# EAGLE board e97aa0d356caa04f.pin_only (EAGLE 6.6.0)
REV: D

Size 50.8 x 22.86 mm. Coordinates in mm from the lower left corner, seen from the top.
Outline: 0,20.95 0,1.91 arc90 1.91,0 48.9,0 arc90 50.8,1.91 50.8,20.95 arc90 48.9,22.86 1.91,22.86 arc90 0,20.95
Copper layers (1*16): Top 0.035mm / dielectric 1.5mm / Bottom 0.035mm
Design rules "adafruit *": minimum track width 10mil, minimum drill 15.5mil, track to track 8mil, track to pad 8mil, pad to pad 8mil, via to via 8mil, smd to smd 8mil, copper to edge 10mil, drill to drill 8mil, minimum pad ring 10mil, minimum via ring 8mil, stop-mask expansion 2mil, vias tented up to drill 20mil, thermal gap 10mil

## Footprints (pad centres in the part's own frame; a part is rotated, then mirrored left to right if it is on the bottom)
0805-NO = smd 1.3 x 1.5: 1 -0.95,0; 2 0.95,0
0805_10MGAP = smd 1.2 x 1.5: 1 -1.05,0; 2 1.05,0
1X14-CB = drill 1.016 pad 1.778: 1 -16.51,0; 2 -13.97,0; 3 -11.43,0; 4 -8.89,0; 5 -6.35,0; 6 -3.81,0; 7 -1.27,0; 8 1.27,0; 9 3.81,0; 10 6.35,0; 11 8.89,0; 12 11.43,0; 13 13.97,0; 14 16.51,0
SOD-323 = smd 1.35 x 0.8: A 1.27,0; C -1.27,0
SOD-123 = smd 1.4 x 1.4: A 1.85,0; C -1.85,0
_0805MP = smd 1.2 x 1.3: 1 -1.016,0; 2 1.016,0
FIDUCIAL_1MM = smd 1 x 1: 1 0,0
CHIPLED_0805_NOOUTLINE = smd 1.2 x 1.2: A 0,-1.05; C 0,1.05
TERMBLOCK_1X2-3.5MM = drill 1 pad 2.184: 1 1.8,0; 2 -1.7,0
RESPACK_4X0603 = smd 0.45 x 0.9: 1 -1.3,-0.85; 2 -0.4,-0.85; 3 0.4,-0.85; 4 1.3,-0.85; 5 1.3,0.85; 6 0.4,0.85; 7 -0.4,0.85; 8 -1.3,0.85
SOLDERJUMPER_ARROW_NOPASTE = smd 0.762 x 1.524: 1 -1.016,0; 2 1.016,0
SOLDERJUMPER_CLOSEDWIRE = smd 1.168 x 1.6: 1 -0.762,0; 2 0.762,0 | smd 0.635 x 0.203: WIRE 0,0
B1,27 = smd 1.27 x 1.27: TP 0,0
SOIC8_208MIL = smd 0.6 x 2.2: 1 -1.905,-3.315; 2 -0.635,-3.315; 3 0.635,-3.315; 4 1.905,-3.315; 5 1.905,3.315; 6 0.635,3.315; 7 -0.635,3.315; 8 -1.905,3.315
LQFP48 = smd 1.1 x 0.285: 1 -4.2,2.75; 2 -4.2,2.25; 3 -4.2,1.75; 4 -4.2,1.25; 5 -4.2,0.75; 6 -4.2,0.25; 7 -4.2,-0.25; 8 -4.2,-0.75; 9 -4.2,-1.25; 10 -4.2,-1.75; 11 -4.2,-2.25; 12 -4.2,-2.75; 25 4.2,-2.75; 26 4.2,-2.25; 27 4.2,-1.75; 28 4.2,-1.25; 29 4.2,-0.75; 30 4.2,-0.25; 31 4.2,0.25; 32 4.2,0.75; 33 4.2,1.25; 34 4.2,1.75; 35 4.2,2.25; 36 4.2,2.75 | smd 0.285 x 1.1: 13 -2.75,-4.2; 14 -2.25,-4.2; 15 -1.75,-4.2; 16 -1.25,-4.2; 17 -0.75,-4.2; 18 -0.25,-4.2; 19 0.25,-4.2; 20 0.75,-4.2; 21 1.25,-4.2; 22 1.75,-4.2; 23 2.25,-4.2; 24 2.75,-4.2; 37 2.75,4.2; 38 2.25,4.2; 39 1.75,4.2; 40 1.25,4.2; 41 0.75,4.2; 42 0.25,4.2; 43 -0.25,4.2; 44 -0.75,4.2; 45 -1.25,4.2; 46 -1.75,4.2; 47 -2.25,4.2 | smd 0.28 x 1.1: 48 -2.75,4.2
WQFN20 = smd 0.28 x 0.75: 1 -1,-1.975; 2 -0.5,-1.975; 3 0,-1.975; 4 0.5,-1.975; 5 1,-1.975; 11 1,1.975; 12 0.5,1.975; 13 0,1.975; 14 -0.5,1.975; 15 -1,1.975 | smd 0.75 x 0.28: 6 1.975,-1; 7 1.975,-0.5; 8 1.975,0; 9 1.975,0.5; 10 1.975,1; 16 -1.975,1; 17 -1.975,0.5; 18 -1.975,0; 19 -1.975,-0.5; 20 -1.975,-1 | smd 2.45 x 2.45: 21 0,0
MOUNTINGHOLE_2.5_PLATED = drill 2.5 pad 3.2: P$1 0,0
4UCONN_20329 = smd 1 x 2: BASE@1 -0.75,-2; BASE@2 0.75,-2 | smd 0.4 x 1.35: D+ 0,0.775; D- -0.65,0.775; GND 1.3,0.775; ID 0.65,0.775; VBUS -1.3,0.775 | drill 0.7 offset: SPRT@1 -3.3,0.9; SPRT@2 3.3,0.9 | drill 0.6 pad 2.5 square: SPRT@3 -3.6,-1.9; SPRT@4 3.6,-1.9 | hole 0.7: -1.95,0; 1.95,0
JSTPH2 = smd 1 x 4.6: 1 -1,-3.7; 2 1,-3.7 | smd 1.6 x 3.4: NC1 -3.4,1.5; NC2 3.4,1.5
RESONATOR-SMD = smd 0.7 x 1.7: 1 -1.2,0; 2 0,0; 3 1.2,0

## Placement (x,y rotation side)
C1  10uF  [0805-NO]  39.75,7.24 270 top
C2  10uF  [0805_10MGAP]  36.7,16 180 top
C3  1uF  [0805-NO]  9.91,10.29 180 top
C4  10µF  [0805-NO]  42.55,7.75 180 top
C5  0.1µF  [0805-NO]  42.04,17.4 180 top
C6  10uF  [0805_10MGAP]  15.37,18.29 180 top
C7  10uF  [0805_10MGAP]  10.92,7.62 270 top
C8  10uF  [0805-NO]  9.65,13.08 90 top
C9  10uF  [0805-NO]  11.18,17.78 270 top
C10  1uF  [0805-NO]  9.27,17.65 270 top
C11  4.7nF  [0805-NO]  40.64,4.19 0 top
C12  4.7nF  [0805-NO]  36.45,17.91 0 top
C13  0.1µF  [0805-NO]  36.58,10.92 0 top
C14  0.1µF  [0805-NO]  42.55,5.97 180 top
C15  1µF  [0805-NO]  36.58,9.14 0 top
C18  1µF  [0805-NO]  36.7,14.22 0 top
CONTROL  Control Breakout  [1X14-CB]  24.13,21.59 0 top
D2  1N4148  [SOD-323]  19.3,18.03 180 top
D3  MBR120  [SOD-123]  5.21,19.56 90 top
D4  MBR120  [SOD-123]  6.86,15.11 270 top
FB1  ferrite  [_0805MP]  42.04,19.05 0 top
FB2  ferrite  [_0805MP]  36.7,12.57 0 top
FID1  FIDUCIAL""  [FIDUCIAL_1MM]  44.45,1.02 0 top
FID2  FIDUCIAL""  [FIDUCIAL_1MM]  0.76,17.91 0 top
GPIO1  GPIO breakout  [1X14-CB]  24.13,1.27 180 top
GREEN  RED  [CHIPLED_0805_NOOUTLINE]  28.32,15.75 90 top
J1  3.5mm  [TERMBLOCK_1X2-3.5MM]  48.64,7.75 90 top
J2  3.5mm  [TERMBLOCK_1X2-3.5MM]  48.64,14.86 90 top
LED4  Green  [CHIPLED_0805_NOOUTLINE]  2.54,5.33 90 top
R1  1M  [0805-NO]  25.15,17.02 270 top
R2  100K  [RESPACK_4X0603]  8,5.84 0 top
R3  470  [0805-NO]  37.97,5.46 270 top
R4  100K  [0805-NO]  44.45,2.79 0 top
R5  100K  [0805-NO]  43.94,20.7 180 top
R6  470  [0805-NO]  33.02,18.29 0 top
R7  470  [0805-NO]  5.08,2.29 90 top
R8  470  [0805-NO]  28.19,17.53 0 top
R9  100K  [RESPACK_4X0603]  14.86,4.95 180 top
R10  100K  [RESPACK_4X0603]  19.43,4.95 180 top
R11  100K  [RESPACK_4X0603]  32.51,7.11 0 top
R12  100K  [RESPACK_4X0603]  27.18,7.11 180 top
SJ1  [SOLDERJUMPER_ARROW_NOPASTE]  43.81,2.16 90 bottom
SJ2  [SOLDERJUMPER_CLOSEDWIRE]  44.7,20.95 270 bottom
TP1  PTR1B1,27  [B1,27]  31.24,11.3 0 bottom
TP2  PTR1B1,27  [B1,27]  22.61,14.86 0 bottom
TP3  PTR1B1,27  [B1,27]  27.81,11.43 0 bottom
U1  MX25L1606  [SOIC8_208MIL]  29.72,11.94 90 top
U2  VS1000  [LQFP48]  16.76,11.94 90 top
U3  TS2012  [WQFN20]  42.29,12.45 0 top
U$5  MOUNTINGHOLE2.5  [MOUNTINGHOLE_2.5_PLATED]  2.16,20.7 0 top
U$6  MOUNTINGHOLE2.5  [MOUNTINGHOLE_2.5_PLATED]  2.16,2.16 0 top
U$7  MOUNTINGHOLE2.5  [MOUNTINGHOLE_2.5_PLATED]  48.64,20.7 0 top
U$8  MOUNTINGHOLE2.5  [MOUNTINGHOLE_2.5_PLATED]  48.64,2.16 0 top
U$11  [ADAFRUIT_2.5MM]  23.62,5.59 90 top
U$12  [SYMBOL_PLUS]  9.14,8.51 0 bottom
U$13  [SYMBOL_MINUS]  9.14,14.35 0 bottom
U$14  [ADAFRUIT_TEXT_20MM]  44.7,12.57 0 bottom
U$15  [PCBFEAT-REV-040]  35.81,6.35 0 top
X1  Micro B  [4UCONN_20329]  4.32,11.43 270 top
X2  JST-PH  [JSTPH2]  3.56,11.43 270 bottom
Y2  12MHz  [RESONATOR-SMD]  22.99,17.14 270 top

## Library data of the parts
C1-C15 C18 D2-D4 FB1 FB2 GREEN J1 J2 LED4 R1-R12 SJ2 U1-U3 U$11-U$15 X1 X2 = microbuilder
CONTROL GPIO1 = adafruit
FID1 FID2 SJ1 U$5-U$8 = microbuilder; BOM: EXCLUDE
TP1-TP3 = testpad
Y2 = SparkFun

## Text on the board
tPlace: Vin | Gnd | PB | TX | RX | UG | + | Vol | - | CS | Gnd | R | L | Gnd | BUS | + | Act | R | - | 2x2W Amp | - | adafruit | L | + | Pwr | 0 | 1 | Sound Board | Rst | 2 | 3 | 4 | 10 | Act | Gnd | 5 | 6 | 7 | 8 | 9
bPlace: G0 | Adafruit Audio FX Sound Board | Vin:3-5VDC | 2W Class D Amp | + | 4-8Ω Speakers | R | - | Vin / JST | 11 GPIO / Triggers / or UART | - | Pin to GND / For Trigger | L | + | WAV or OGG / Stereo Files | T00.WAV / T01HOLDL.OGG / T02LATCH.WAV / T03RAND0.OGG..T03RAND9.OGG / T04NEXT0.WAV..T04NEXT9.WAV / ... -> T10.WAV | G1

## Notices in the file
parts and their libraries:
microbuilder: This work is placed in the public domain, and may be freely used for commercial and non-commercial work with the following conditions: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
SparkFun: Licensing: CC v3.0 Share-Alike You are welcome to use this library for commercial purposes.
